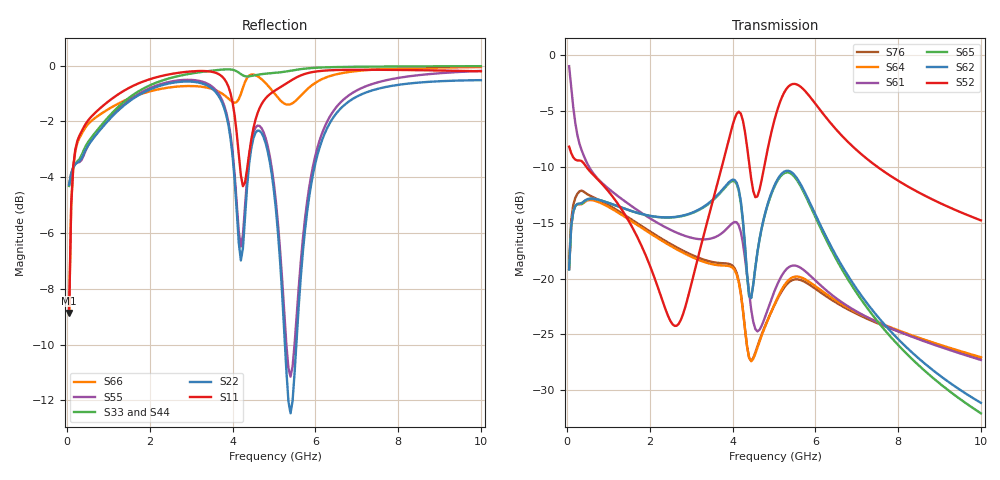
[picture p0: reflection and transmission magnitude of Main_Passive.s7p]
! Created Fri Dec 28 22:59:16 2018
# ghz S ma R 50
! 7 Port Network Data from SP1.SP block
! freq  magS11  angS11  magS12  angS12  magS13  angS13  magS14  angS14
!  magS15  angS15  magS16  angS16  magS17  angS17
!  magS21  angS21
!  magS22  angS22  magS23  angS23  magS24  angS24  magS25  angS25
!  magS26  angS26  magS27  angS27
!  magS31  angS31  magS32  angS32
!  magS33  angS33  magS34  angS34  magS35  angS35  magS36  angS36
!  magS37  angS37
!  magS41  angS41  magS42  angS42  magS43  angS43
!  magS44  angS44  magS45  angS45  magS46  angS46  magS47  angS47
!  magS51  angS51  magS52  angS52  magS53  angS53  magS54  angS54
!  magS55  angS55  magS56  angS56  magS57  angS57
!  magS61  angS61
!  magS62  angS62  magS63  angS63  magS64  angS64  magS65  angS65
!  magS66  angS66  magS67  angS67
!  magS71  angS71  magS72  angS72
!  magS73  angS73  magS74  angS74  magS75  angS75  magS76  angS76
!  magS77  angS77
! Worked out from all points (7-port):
!   200 points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, 50 MHz to 10 GHz, reference 50 ohm
!   strongest paths, dB at 50 MHz, 2.55 GHz, 5.05 GHz, 7.55 GHz, 10 GHz:
!     S52: -8.2, -24.1, -5.3, -10.1, -14.8
!     S62: -19.2, -14.5, -11.4, -23.6, -31.1
!     S65: -19.2, -14.5, -11.5, -24.1, -32.1
!     S61: -1.0, -15.7, -20.8, -24.0, -27.3
!     S64: -19.2, -17.2, -22.0, -24.0, -27.1
!     S76: -18.7, -17.0, -22.1, -24.1, -27.1
!   lowest |S11| = -8.9 dB at 50 MHz (marker M1), VSWR 2.13, Z = 29.9 - j22.1 ohm
!   |S11| at or under -10 dB: nowhere
